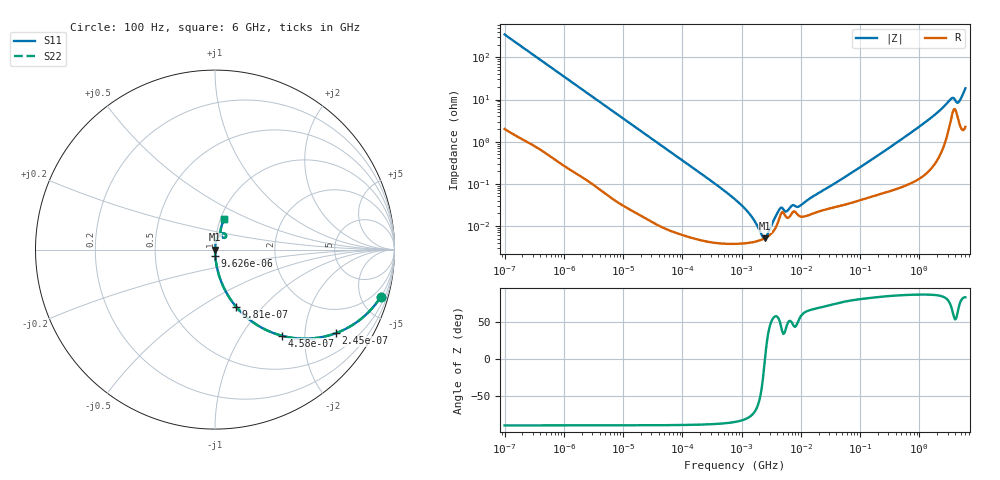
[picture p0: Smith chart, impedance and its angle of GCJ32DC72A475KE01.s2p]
!Murata Part Number: GCJ32DC72A475KE01
!These Parameters are Measured in Series Mode Connection
!Data Generated on Mar 13, 2026
!  o--ll--o
!Port1  Port2
!  o------o
!Operation Temp=25[degC], DC Bias Voltage=0[V]
!Freq. Start=100[Hz] Stop=6[GHz] 401[Steps]
# Hz S RI R 50
!Freq.(Hz) S11(Real) S11(Imag) S21(Real) S21(Imag) S12(Real) S12(Imag) S22(Real) S22(Imag)
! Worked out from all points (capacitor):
!   401 points, 100 Hz to 6 GHz, reference 50 ohm
!   read as one part in series: C = 4.54 uF near 109 Hz
!   lowest |Z| = 5.12 mohm at 2.481 MHz (marker M1)
!   series resonance near 2.485 MHz, so ESL is about 900 pH
!   S11 on the Smith chart (normalised r, x): 100 Hz: 1.04, -7.00; 245 Hz: 1.02, -2.87; 458 Hz: 1.01, -1.54; 981 Hz: 1.01, -0.72; 9.626 kHz: 1.00, -0.07; 6 GHz: 1.04, +0.37
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100  0.9232 -0.2634  0.0768 0.2634  0.0768 0.2634  0.9232 -0.2634
245  0.6716 -0.4663  0.3284 0.4663  0.3284 0.4663  0.6716 -0.4663
458  0.3722 -0.4797  0.6278 0.4797  0.6278 0.4797  0.3722 -0.4797
981  0.1167 -0.3173  0.8833 0.3173  0.8833 0.3173  0.1167 -0.3173
2008  0.0316 -0.1708  0.9684 0.1708  0.9684 0.1708  0.0316 -0.1708
9626  0.00169 -0.0371  0.9983 0.0371  0.9983 0.0371  0.00169 -0.0371
40335  0.000181 -0.00892  0.9998 0.00892  0.9998 0.00892  0.000181 -0.00892
774597  3.76e-05 -0.000426  1 0.000426  1 0.000426  3.76e-05 -0.000426
1212075  3.9e-05 -0.000231  1 0.000231  1 0.000231  3.9e-05 -0.000231
1813585  4.32e-05 -9.58e-05  1 9.58e-05  1 9.58e-05  4.32e-05 -9.58e-05
2481164  5.12e-05 -5e-07  0.9999 5e-07  0.9999 5e-07  5.12e-05 -5e-07
3103719  6.37e-05 7.11e-05  0.9999 -7.11e-05  0.9999 -7.11e-05  6.37e-05 7.11e-05
4440638  0.000166 0.000196  0.9998 -0.000196  0.9998 -0.000196  0.000166 0.000196
5809218  0.000157 0.000158  0.9998 -0.000158  0.9998 -0.000158  0.000157 0.000158
7266822  0.000211 0.000228  0.9998 -0.000228  0.9998 -0.000228  0.000211 0.000228
9506416  0.000171 0.00024  0.9998 -0.00024  0.9998 -0.00024  0.000171 0.00024
1.555665e7  0.000194 0.000447  0.9998 -0.000447  0.9998 -0.000447  0.000194 0.000447
3.124326e8  0.000712 0.00716  0.9993 -0.00716  0.9993 -0.00716  0.000712 0.00716
1.497423e9  0.00328 0.0346  0.9967 -0.0346  0.9967 -0.0346  0.00328 0.0346
3.352442e9  0.0367 0.0901  0.9633 -0.0901  0.9633 -0.0901  0.0367 0.0901
4.586474e9  0.0367 0.0741  0.9633 -0.0741  0.9633 -0.0741  0.0367 0.0741
6e9  0.0526 0.1704  0.9474 -0.1704  0.9474 -0.1704  0.0526 0.1704
